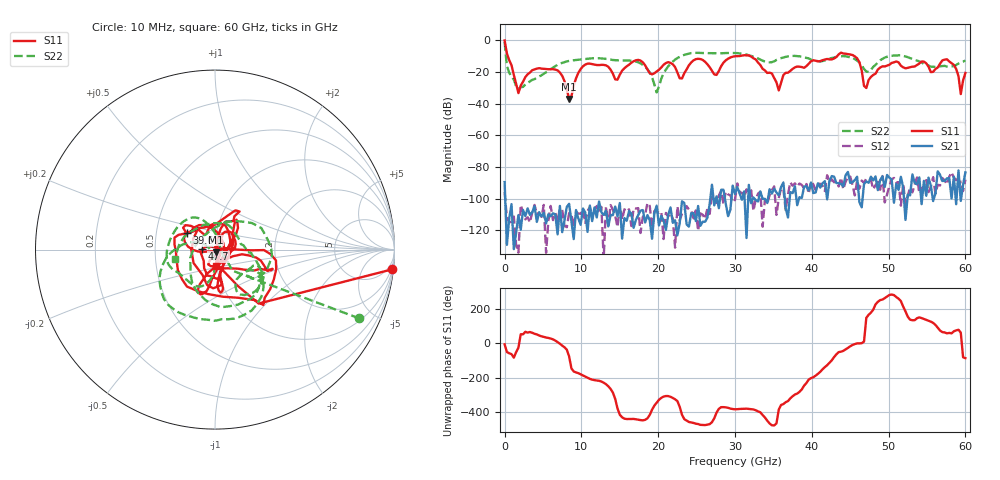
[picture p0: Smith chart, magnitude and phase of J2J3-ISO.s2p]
!Keysight Technologies,N5227A,US51270214,A.10.65.11
!Date: Thursday, October 15, 2020 08:11:33
!Correction: S11(Full 2 Port(1,2))
!S21(Full 2 Port(1,2))
!S12(Full 2 Port(1,2))
!S22(Full 2 Port(1,2))
!S2P File: Measurements: S11, S21, S12, S22:
# Hz S  dB  R 50
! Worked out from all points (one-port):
!   201 points, 10 MHz to 60 GHz, reference 50 ohm
!   lowest |S11| = -37.0 dB at 8.409 GHz (marker M1), VSWR 1.03, Z = 50.3 - j1.38 ohm
!   |S11| at or under -10 dB: 433.5 MHz to 30.19 GHz (29.75 GHz wide, 194 % of centre); 32.01 GHz to 43.3 GHz (11.28 GHz wide, 30 % of centre); 45.56 GHz to end of sweep
!   S11 on the Smith chart (normalised r, x): 10 MHz: 1, -18; 39.6 GHz: 0.72, +0.14; 47.7 GHz: 0.87, +0.01; 60 GHz: 0.99, -0.19
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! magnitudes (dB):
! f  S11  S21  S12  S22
! 10 MHz  0.0  -89.6  -95.9  -1.0
! 309.9 MHz  -8.2  -129.2  -112.3  -16.3
! 1.81 GHz  -33.3  -110.4  -134.1  -30.8
! 6.309 GHz  -18.2  -109.3  -113.6  -17.1
! 8.409 GHz  -37.0  -103.3  -109.1  -13.0
! 10.21 GHz  -16.4  -106.2  -106.9  -11.9
! 14.71 GHz  -24.8  -111.2  -118.0  -12.6
! 17.11 GHz  -12.6  -113.3  -106.3  -13.3
! 20.11 GHz  -18.5  -116.9  -109.0  -29.2
! 23.11 GHz  -24.0  -101.7  -109.5  -9.7
! 30 GHz  -10.0  -97.2  -100.8  -8.0
! 35.7 GHz  -31.6  -97.9  -99.6  -11.7
! 39.6 GHz  -14.8  -94.9  -96.9  -11.4
! 40.2 GHz  -12.6  -96.5  -91.0  -12.7
! 45.3 GHz  -9.2  -89.7  -91.4  -10.9
! 46.8 GHz  -28.8  -90.8  -90.1  -18.1
! 47.7 GHz  -23.1  -86.1  -88.2  -18.6
! 50.1 GHz  -15.4  -86.8  -92.1  -9.8
! 57.6 GHz  -11.9  -87.2  -91.0  -16.5
! 58.8 GHz  -18.1  -103.5  -88.0  -15.6
! 59.4 GHz  -33.9  -101.5  -89.2  -13.9
! 60 GHz  -20.6  -83.4  -88.0  -12.7
